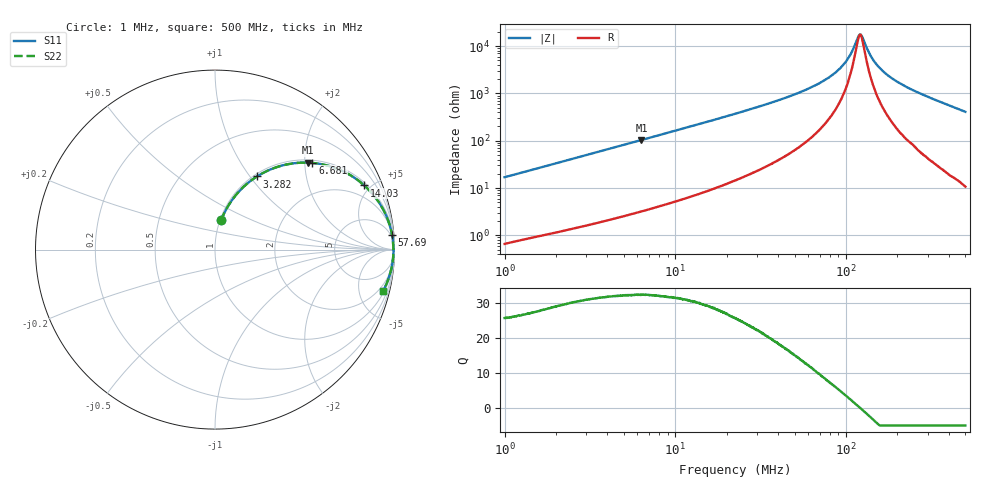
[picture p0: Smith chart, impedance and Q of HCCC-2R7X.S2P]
!s-Parameter Generated by FASTRON Sdn. Bhd.
!FASTRON P/N : HCCC-2R7X
!Keysight Technologies,E4991B,MY54100416,A.01.15
!Date: Mon Apr 06 14:59:15 2026
!Version  : Rev00 Mon Apr 06 14:59:15 2026
!Data & Calibration Information:
!PortZ  Port1:50+j0  Port2:50+j0
!When reading, reference impedance value at option line is always used.
!Remarks : This data is being provided solely for informational purposes.
!Freq	S11	S21	S12	S22
# Hz S dB R 50
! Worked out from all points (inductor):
!   1601 points, 1 MHz to 500 MHz, reference 50 ohm
!   read as one part in series: L = 2.67 uH near 1.032 MHz
!   highest Q = 32.4 at 6.328 MHz (marker M1), where L = 2.6 uH
!   self-resonance near 120.7 MHz
!   S11 on the Smith chart (normalised r, x): 1 MHz: 1.01, +0.34; 3.282 MHz: 1.03, +1.08; 6.681 MHz: 1.07, +2.18; 14.03 MHz: 1.15, +4.58; 57.69 MHz: 3, +23; 500 MHz: 1.21, -8.16
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1000000  -15.61 78.2  -0.18 -9.5  -0.18 -9.5  -15.61 78.2
1769978  -11.04 71.7  -0.45 -16.3  -0.45 -16.3  -11.04 71.7
2820919  -7.59 63.5  -0.96 -24.7  -0.96 -24.7  -7.59 63.5
3282298  -6.56 60.2  -1.23 -28.0  -1.23 -28.0  -6.56 60.2
6327858  -3.00 43.2  -3.29 -45.0  -3.29 -45.0  -3.00 43.2
6681481  -2.78 41.7  -3.54 -46.5  -3.54 -46.5  -2.78 41.7
7957584  -2.15 36.9  -4.42 -51.3  -4.42 -51.3  -2.15 36.9
1.403015e7  -0.86 23.3  -8.06 -64.8  -8.06 -64.8  -0.86 23.3
2.236068e7  -0.39 14.9  -11.77 -72.8  -11.77 -72.8  -0.39 14.9
5.7687e7  -0.09 4.8  -21.51 -80.7  -21.51 -80.7  -0.09 4.8
6.307767e7  -0.08 4.1  -22.78 -80.8  -22.78 -80.8  -0.08 4.1
7.963189e7  -0.06 2.6  -26.88 -79.7  -26.88 -79.7  -0.06 2.6
9.374216e7  -0.05 1.5  -31.18 -76.3  -31.18 -76.3  -0.05 1.5
1.045122e8  -0.05 0.9  -35.69 -68.6  -35.69 -68.6  -0.05 0.9
1.16973e8  -0.05 0.2  -43.50 -31.7  -43.50 -31.7  -0.05 0.2
1.206648e8  -0.05 0.0  -44.95 -2.6  -44.95 -2.6  -0.05 0.0
1.244731e8  -0.05 -0.2  -43.82 27.6  -43.82 27.6  -0.05 -0.2
1.361047e8  -0.05 -0.7  -37.33 65.4  -37.33 65.4  -0.05 -0.7
1.459609e8  -0.05 -1.1  -33.68 73.2  -33.68 73.2  -0.05 -1.1
1.77937e8  -0.06 -2.4  -27.41 80.0  -27.41 80.0  -0.06 -2.4
2.583476e8  -0.09 -5.2  -20.78 81.1  -20.78 81.1  -0.09 -5.2
5e8  -0.31 -13.7  -12.52 74.8  -12.52 74.8  -0.31 -13.7
